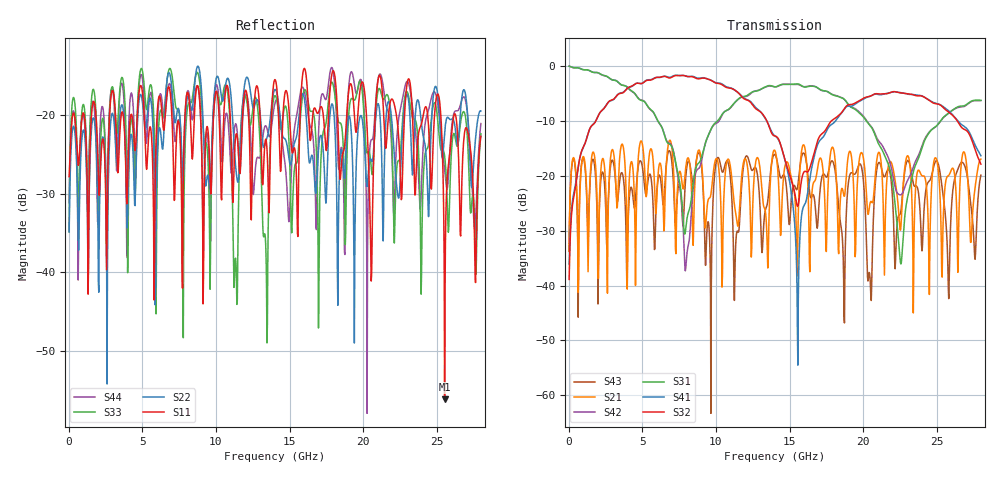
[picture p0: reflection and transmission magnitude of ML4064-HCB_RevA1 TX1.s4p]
! TOUCHSTONE file generated by CST DESIGN STUDIO
! Date and time: Wed Aug 26 10:46:48 2020
! Project name:  Project name: C:\Users\Simulation2\Temp\DE66\Untitled_0.cst
! Tree item: Tasks\SPara1\S-Parameters
# GHz S MA R 50
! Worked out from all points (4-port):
!   1000 points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, 28 MHz to 28 GHz, reference 50 ohm
!   strongest paths, dB at 28 MHz, 7.028 GHz, 14.03 GHz, 21.03 GHz, 28 GHz:
!     S32: -38.9, -2.1, -12.8, -5.1, -17.9
!     S41: -36.1, -1.9, -12.8, -5.2, -16.4
!     S31: -0.1, -14.9, -3.8, -14.1, -6.3
!     S42: -0.1, -14.7, -3.8, -13.6, -6.3
!     S21: -33.8, -15.4, -15.6, -15.9, -17.0
!     S43: -33.7, -18.1, -16.2, -17.7, -19.9
!   lowest |S11| = -56.1 dB at 25.54 GHz (marker M1), VSWR 1.00, Z = 49.9 - j0.123 ohm
!   |S11| at or under -10 dB: start of sweep to end of sweep
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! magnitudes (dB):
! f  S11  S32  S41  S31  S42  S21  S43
! 28 MHz  -27.9  -38.9  -36.1  -0.1  -0.1  -33.8  -33.7
! 7.98 GHz  -18.0  -1.9  -1.9  -29.0  -35.8  -17.9  -19.4
! 14.25 GHz  -20.1  -13.3  -13.5  -3.6  -3.7  -21.1  -18.7
! 15.57 GHz  -35.4  -25.6  -54.5  -3.3  -3.4  -30.9  -21.8
! 22.54 GHz  -28.1  -4.9  -4.9  -35.9  -23.5  -29.9  -26.8
! 25.54 GHz  -56.1  -7.9  -7.6  -9.2  -9.2  -22.8  -25.9
! 28 GHz  -22.8  -17.9  -16.4  -6.3  -6.3  -17.0  -19.9
